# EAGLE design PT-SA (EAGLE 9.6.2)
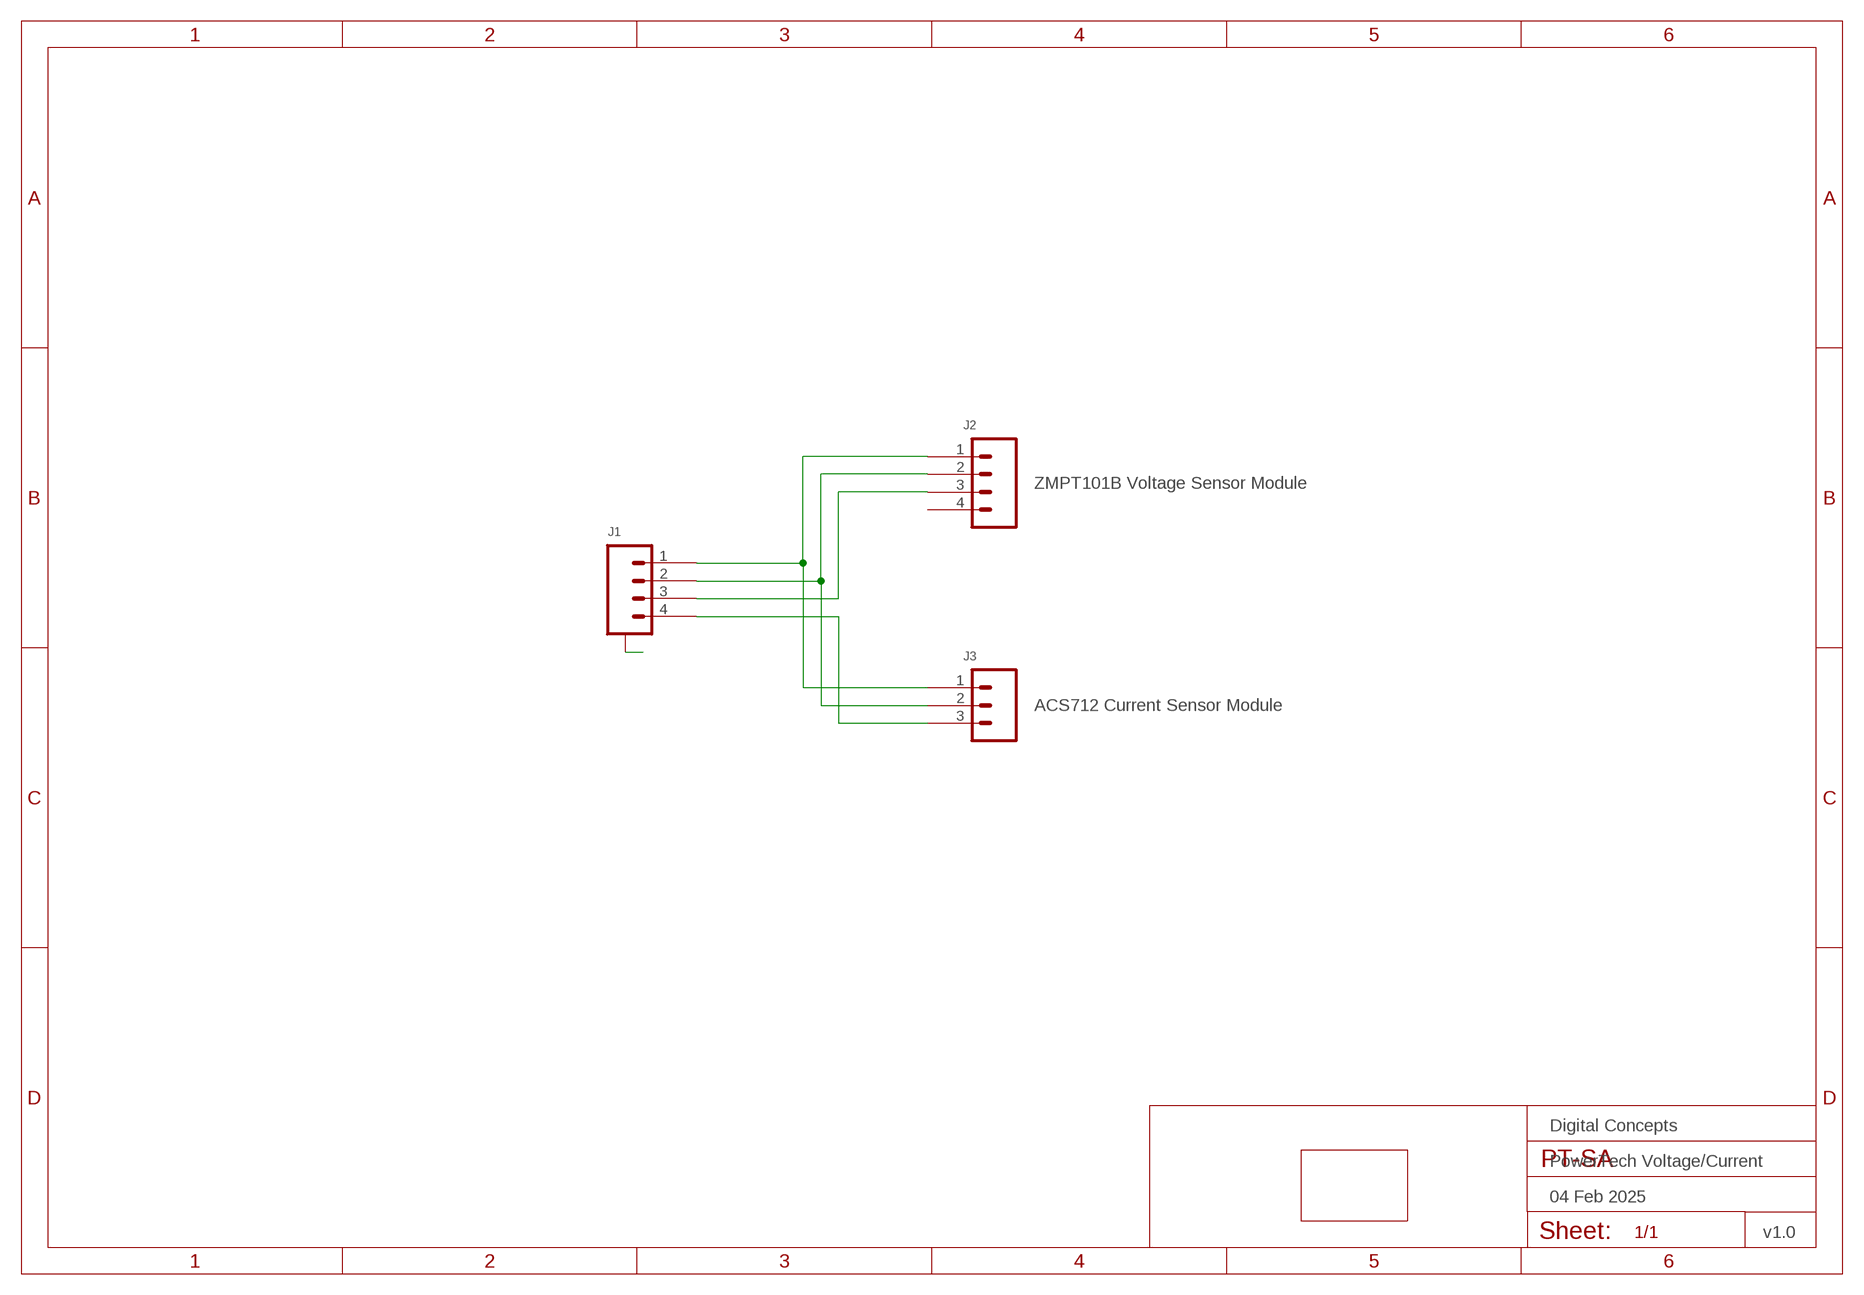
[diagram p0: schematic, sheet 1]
FRAME2 (FRAME-A4L-LOC): DATE: 04 Feb 2025; OWNER: Digital Concepts; TITLE: PowerTech Voltage/Current; VERSION: v1.0

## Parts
J1  JST-SH1.0-4-SMD-HORIZONTAL  [JST-SH1.0-4-HORIZONTAL]
J2  ZMPT101B Voltage Sensor Module  HEADER-1X4-GENERIC  [CONN_04-GENERIC]
J3  ACS712 Current Sensor Module  HEADER-1X3-GENERIC  [CONN_03-GENERIC]
PCB1  POWERTECH-SOCKET  [PCB-POWERTECH]

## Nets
A: J1.A@1(A) J1.A@4(A)
N$1: J1.1 J2.1 J3.1
N$2: J1.2 J2.2 J3.2
N$3: J1.3 J2.3
N$4: J1.4 J3.3
Unconnected: J2.4

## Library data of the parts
J1 = digitalconcepts:JST-SH1.0-4-SMD-HORIZONTAL: JST SH1.0 4P SMD horizontal connector
J2 = digitalconcepts:HEADER-1X4-GENERIC: Single Row 4-Pin Header
J3 = digitalconcepts:HEADER-1X3-GENERIC: Single Row 3-Pin Header
PCB1 = digitalconcepts:POWERTECH-SOCKET: PowerTech Socket Outlet Adaptor PCB

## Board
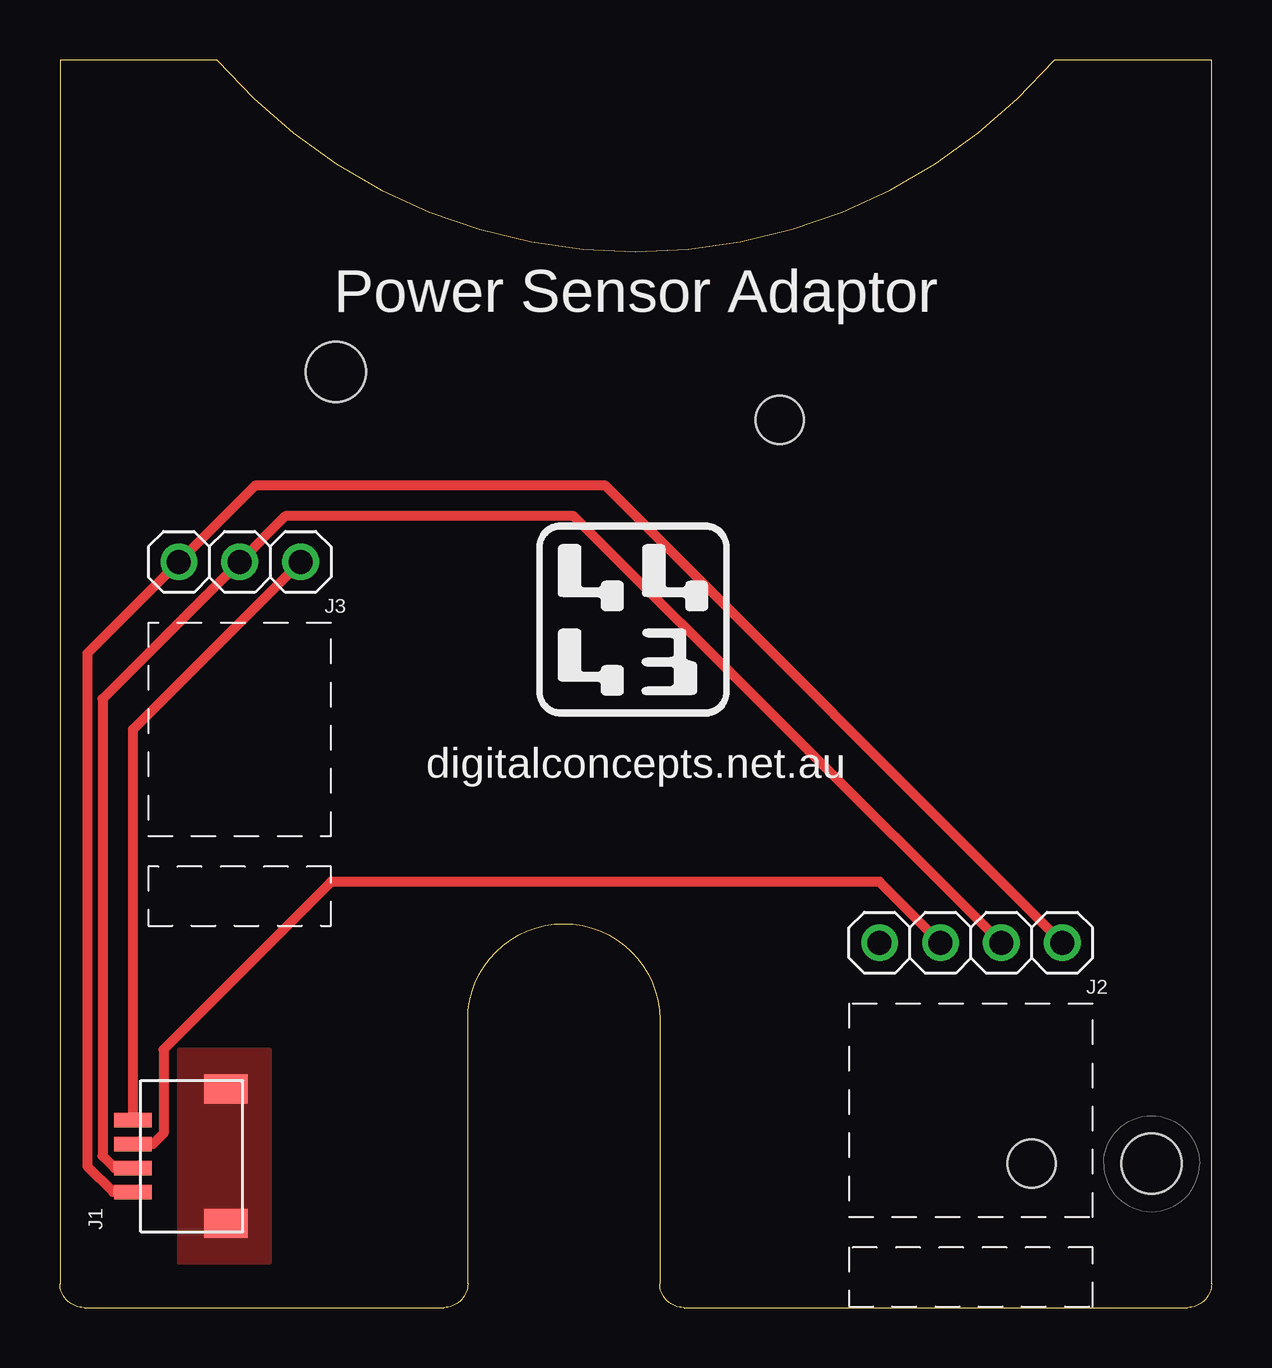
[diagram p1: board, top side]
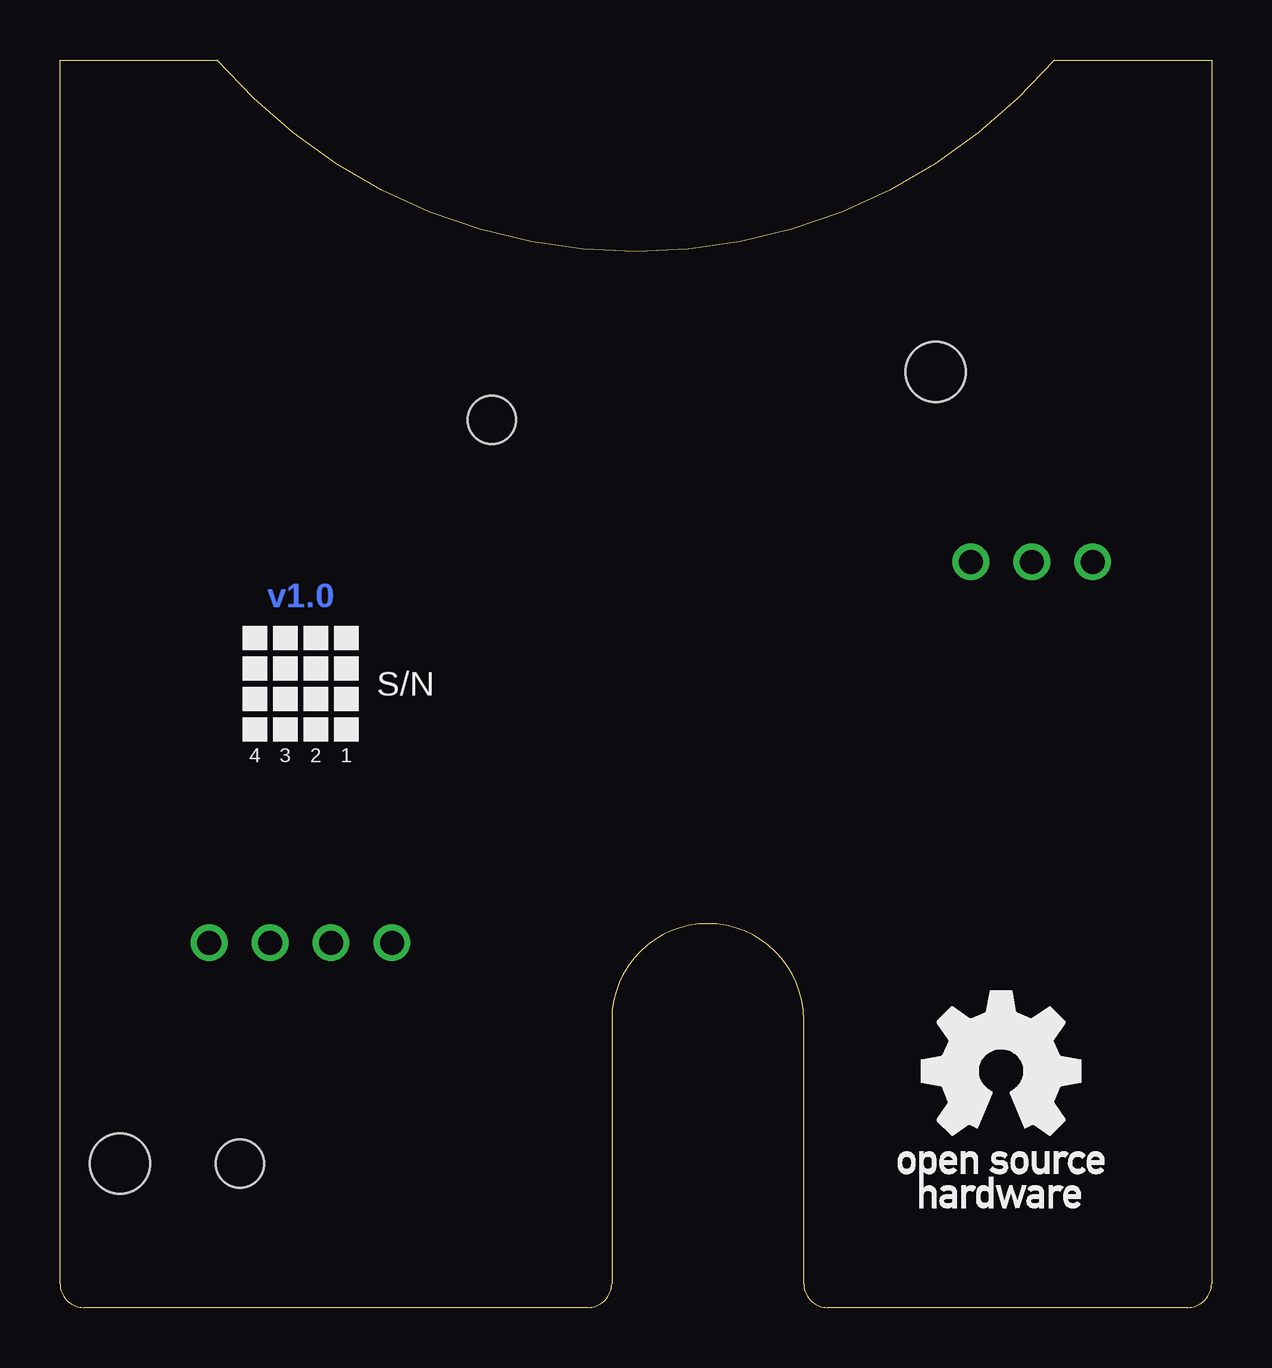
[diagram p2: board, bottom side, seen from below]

Size 48 x 52 mm. Coordinates in mm from the lower left corner, seen from the top.
Copper layers (1*16): Top 0.035mm / dielectric 1.5mm / Bottom 0.035mm
Design rules "default *": minimum track width 6mil, minimum drill 0.35mm, track to track 6mil, track to pad 6mil, pad to pad 6mil, via to via 6mil, smd to smd 6mil, copper to edge 6mil, drill to drill 6mil, minimum pad ring 10mil, minimum via ring 8mil, stop-mask expansion 4mil, vias tented up to drill 0mil, thermal gap 10mil

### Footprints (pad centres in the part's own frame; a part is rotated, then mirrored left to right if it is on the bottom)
JST-SH1.0-4-HORIZONTAL = smd 0.6 x 1.55: 1 -1.5,2.54; 2 -0.5,2.54; 3 0.5,2.54; 4 1.5,2.54 | smd 1.2 x 1.8: A@1 -2.8,-1.335; A@4 2.8,-1.335
CONN_04-GENERIC = drill 1 pad 1.524: 1 0,0; 2 2.54,0; 3 5.08,0; 4 7.62,0
CONN_03-GENERIC = drill 1 pad 1.524: 1 0,0; 2 2.54,0; 3 5.08,0
PCB-POWERTECH = hole 2.5: -20,-21.5; 13,12.5 | hole 2: -20,-16.5; 11,-6

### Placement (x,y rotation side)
J1  5.59,6.31 90 top
J2  41.78,15.2 180 top
J3  4.95,31.08 0 top
PCB1  24,26 90 top

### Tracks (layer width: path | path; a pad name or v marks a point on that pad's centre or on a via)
A
  pour Top (no thermals): 4.95,10.76 8.76,10.76 8.76,1.87 4.95,1.87
N$1
  Top 0.406: J2.1 22.73,34.25 8.13,34.25 J3.1 1.14,27.27 1.14,5.89 2.21,4.81 J1.1
N$2
  Top 0.406: J2.2 21.41,32.98 9.4,32.98 J3.2 1.78,25.36 1.78,6.31 2.28,5.81 J1.2
N$3
  Top 0.406: J2.3 34.16,17.74 11.3,17.74 4.32,10.76 4.32,7.25 3.88,6.81 J1.3
N$4
  Top 0.406: J1.4 3.05,24.09 J3.3

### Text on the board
Bottom: v1.0
tPlace: Power Sensor Adaptor | digitalconcepts.net.au
bPlace: S/N | 1 | 2 | 3 | 4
